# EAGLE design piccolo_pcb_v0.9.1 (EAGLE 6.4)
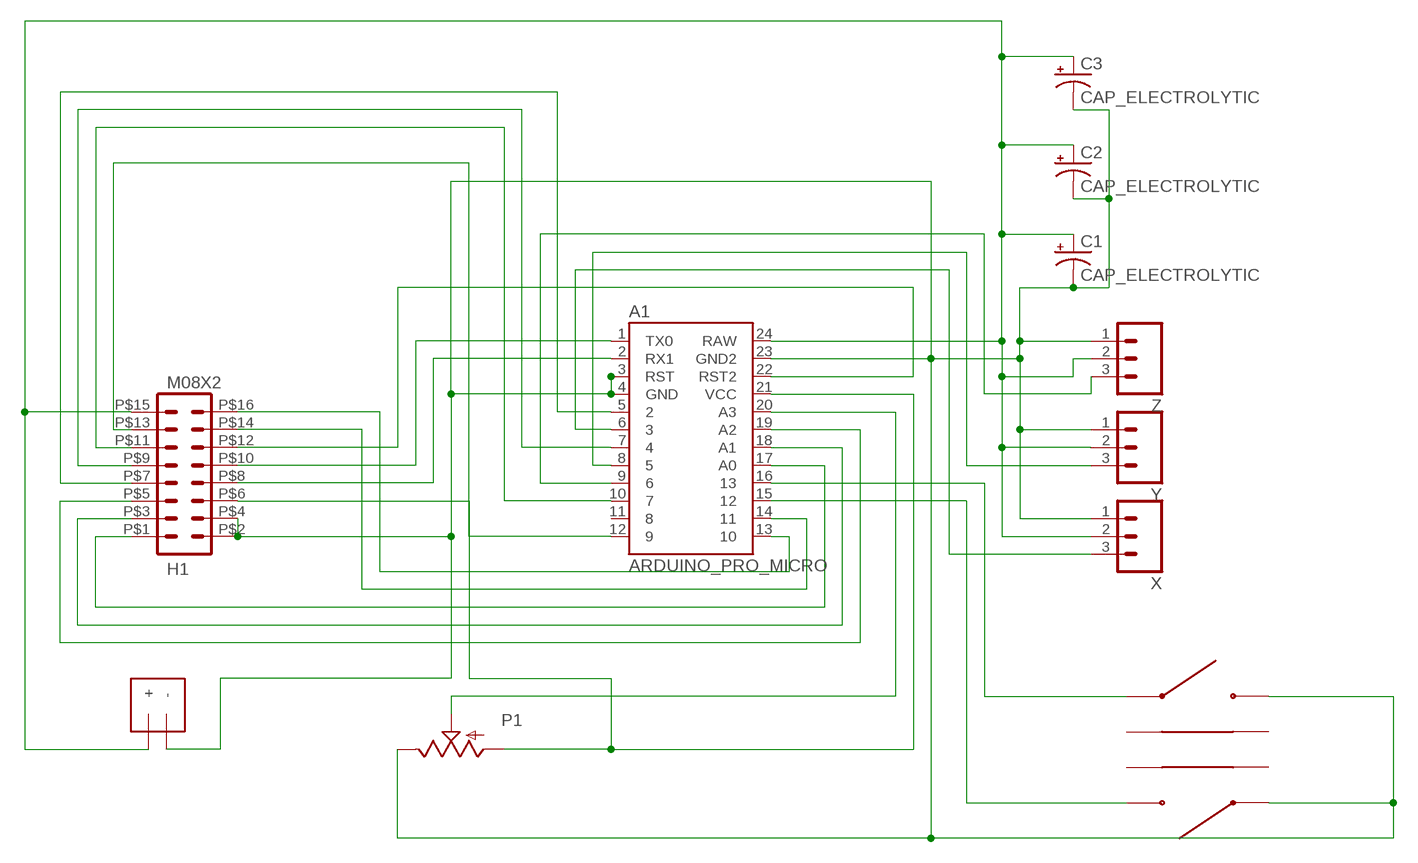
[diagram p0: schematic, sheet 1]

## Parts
A1  ARDUINO_PRO_MICRO  ARDUINO_MINI  [ARDUINO_MINI]
C1  CAP_ELECTROLYTIC  [RADIAL_330UF]
C2  CAP_ELECTROLYTIC  [RADIAL_330UF]
C3  CAP_ELECTROLYTIC  [RADIAL_330UF]
DC_IN  4.8v-6.0v  M02-POL  [JST-PH-2-PTH]
H1  M08X2  [PTH_2X8_90DEG_FEMALE]
P1  POTTHUMBWHEEL  [16MM_THUMBWHEEL]
S1  SWITCH_TACTILE  [RIGHT_ANGLE_TACTSWITCH]
S2  SWITCH_TACTILE  [RIGHT_ANGLE_TACTSWITCH]
X  M03PTH  [1X03]
Y  M03PTH  [1X03]
Z  M03PTH  [1X03]

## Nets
A3: A1.20(A3) P1.P$2(S)
GND: A1.3(RST) A1.4(GND) A1.23(GND2) C1.C(-) C2.C(-) C3.C(-) DC_IN.- H1.P$2 H1.P$4 P1.P$1(E) S1.1 S2.2 X.1 Y.1 Z.1
N$3: A1.15 S1.2
N$4: A1.16 S2.1
PIN2: A1.5 H1.P$7
PIN4: A1.7 H1.P$9
PIN7: A1.10 H1.P$11
PIN9: A1.12 H1.P$13
PIN10: A1.13 H1.P$16
PIN16: A1.14 H1.P$14
PIN_A0: A1.17(A0) H1.P$1
PIN_A1: A1.18(A1) H1.P$3
PIN_A2: A1.19(A2) H1.P$5
PWR_RAW: A1.24(RAW) C1.A(+) C2.A(+) C3.A(+) DC_IN.+ H1.P$15 X.2 Y.2 Z.2
RESET: A1.22(RST2) H1.P$12
RX: A1.2(RX1) H1.P$8
TX: A1.1(TX0) H1.P$10
VCC: A1.21(VCC) H1.P$6 P1.P$3(A)
X_PWM_PIN3: A1.6 X.3
Y_PWM_PIN5: A1.8 Y.3
Z_PWM_PIN6: A1.9 Z.3
Unconnected: A1.11 S1.PE1(GND1) S1.PE2(GND2) S2.PE1(GND1) S2.PE2(GND2)

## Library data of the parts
A1 = SparkFun-Boards:ARDUINO_MINI: Arduino Pro Mini footprint
C1-C3 = Piccolo:CAP_ELECTROLYTIC
DC_IN = Piccolo:M02-POL
H1 = Piccolo:M08X2
P1 = Piccolo:POT
S1 S2 = Piccolo:SWITCH_TACTILE
X Y Z = SparkFun-Connectors:M03: Header 3 Standard 3-pin 0.1" header. Use with straight break away headers (SKU : PRT-00116), right angle break away headers (PRT-00553), swiss pins (PRT-00743), machine pins (PRT-00117), and female headers (PRT-00115). Molex polarized connector foot print use with SKU : PRT-08232 with associated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

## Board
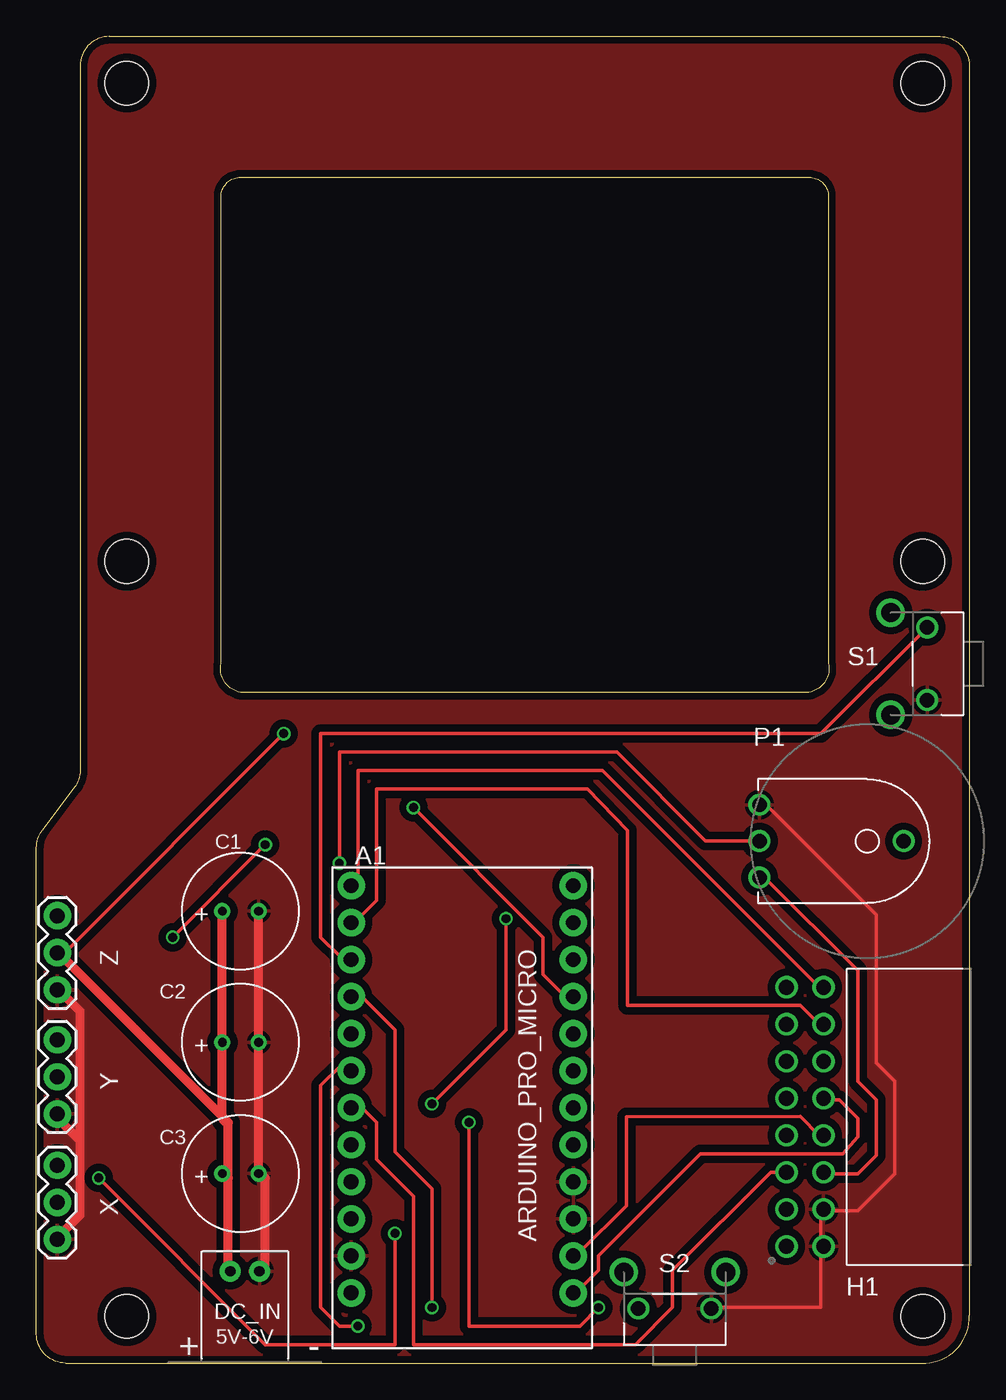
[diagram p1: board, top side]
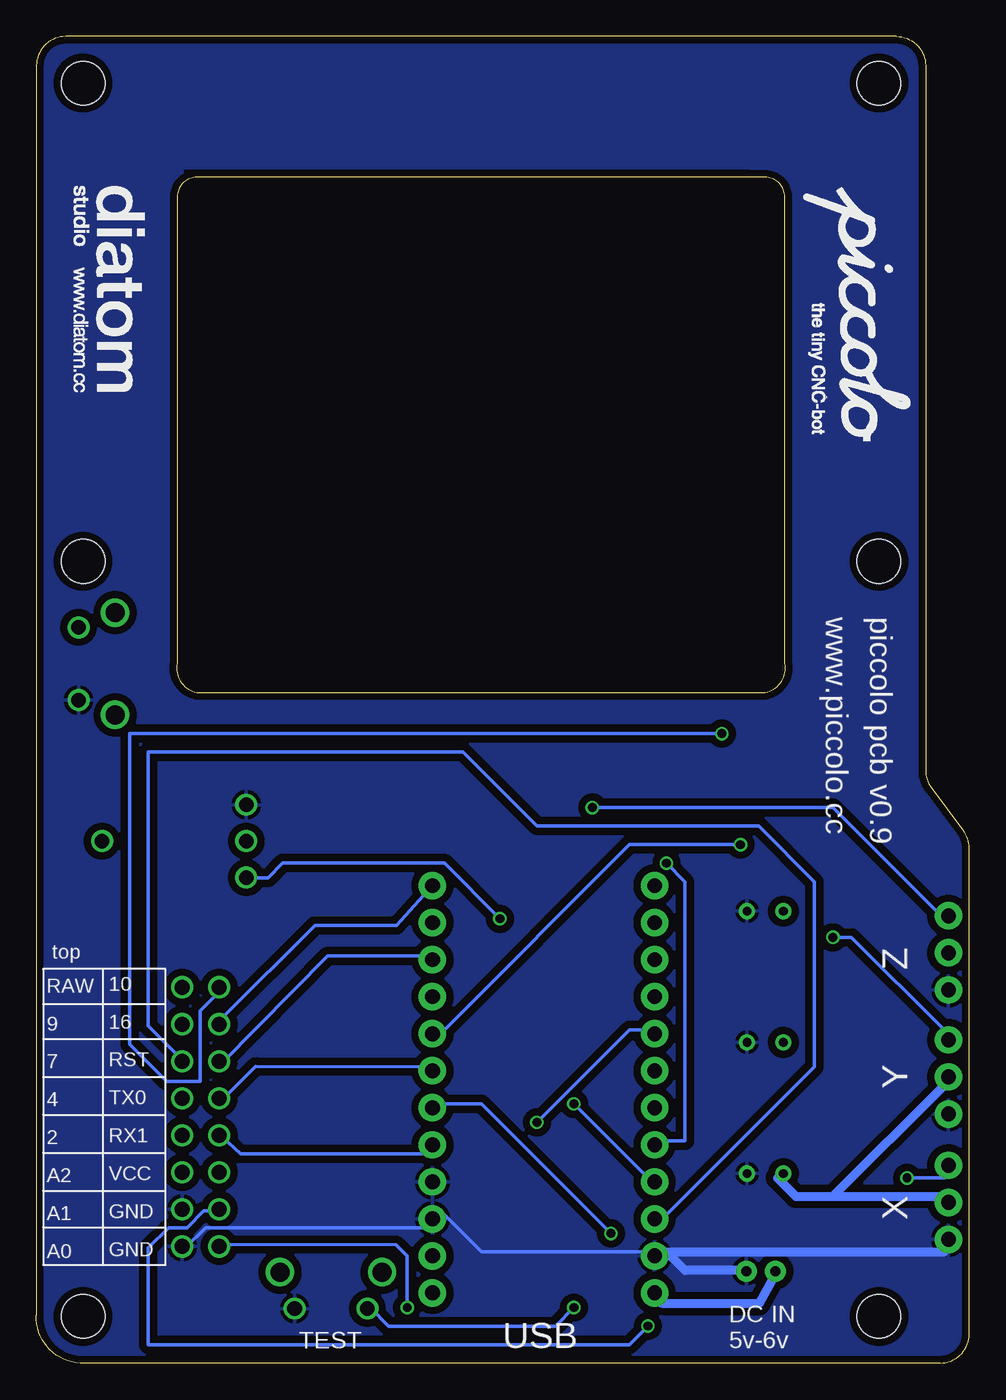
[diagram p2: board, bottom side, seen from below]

Size 64 x 91 mm. Coordinates in mm from the lower left corner, seen from the top.
Outline: 0,2 0,35.33 arc-37 0.4,36.53 2.6,39.47 arc37 3,40.67 3,89 arc-90 5,91 62,91 arc-90 64,89 64,3.27 arc-90 61,0 2,0 arc-90 0,2
Outline: 12.66,48 12.66,80 arc-90 14,81.34 53,81.34 arc-90 54.34,80 54.34,48 arc-90 53,46 14,46 arc-90 12.66,48
Copper layers (1*16): Top 0.035mm / dielectric 1.5mm / Bottom 0.035mm
Design rules "ITEADstudio_DRC": minimum track width 6mil, minimum drill 12mil, track to track 6mil, track to pad 6mil, pad to pad 6mil, via to via 6mil, smd to smd 0mil, copper to edge 10mil, drill to drill 10mil, minimum pad ring 10mil, minimum via ring 6mil, stop-mask expansion 2mil, vias tented up to drill 100mil, thermal gap 10mil
Holes 3 mm at 6.2,87.8 6.2,55 6.2,3.2 60.8,3.2 60.8,55 60.8,87.8

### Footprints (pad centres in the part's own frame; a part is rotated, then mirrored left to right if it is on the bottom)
ARDUINO_MINI = drill 1.016 pad 1.88: 1 -7.62,12.7; 2 -7.62,10.16; 3 -7.62,7.62; 4 -7.62,5.08; 5 -7.62,2.54; 6 -7.62,0; 7 -7.62,-2.54; 8 -7.62,-5.08; 9 -7.62,-7.62; 10 -7.62,-10.16; 11 -7.62,-12.7; 12 -7.62,-15.24; 13 7.62,-15.24; 14 7.62,-12.7; 15 7.62,-10.16; 16 7.62,-7.62; 17 7.62,-5.08; 18 7.62,-2.54; 19 7.62,0; 20 7.62,2.54; 21 7.62,5.08; 22 7.62,7.62; 23 7.62,10.16; 24 7.62,12.7
RADIAL_330UF = drill 0.6: A 0,1.25; C 0,-1.25
JST-PH-2-PTH = drill 0.7 pad 1.448: + -1,0; - 1,0
PTH_2X8_90DEG_FEMALE = drill 1.02: P$1 -2.54,0; P$2 0,0; P$3 -2.54,2.54; P$4 0,2.54; P$5 -2.54,5.08; P$6 0,5.08; P$7 -2.54,7.62; P$8 0,7.62; P$9 -2.54,10.16; P$10 0,10.16; P$11 -2.54,12.7; P$12 0,12.7; P$13 -2.54,15.24; P$14 0,15.24; P$15 -2.54,17.78; P$16 0,17.78
16MM_THUMBWHEEL = drill 1: P$1 -2.5,-7.4; P$2 0,-7.4; P$3 2.5,-7.4; P$4 0,2.5
RIGHT_ANGLE_TACTSWITCH = drill 1: 1 -2.5,0; 2 2.5,0 | drill 1.3: PE1 -3.5,2.5; PE2 3.5,2.5
1X03 = drill 1.016 pad 1.88: 1 0,0; 2 2.54,0; 3 5.08,0

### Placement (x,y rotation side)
A1  29.21,17.51 180 top
C1  14,31 90 top
C2  14,22 90 top
C3  14,13 90 top
DC_IN  14.3,6.3 0 top
H1  54,8 0 top
P1  57,35.8 270 top
S1  61.11,47.97 90 top
S2  43.79,3.74 0 top
X  1.43,8.48 90 top
Y  1.43,17.09 90 top
Z  1.43,25.6 90 top

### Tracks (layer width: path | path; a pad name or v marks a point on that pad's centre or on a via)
A3  (via drill 0.61)
  Top 0.254: v20.78,34.29 20.78,41.91 39.83,41.91 45.91,35.83 49.99,35.83 P1.P$2
  Bottom 0.254: v20.78,34.29 19.51,33.02 19.51,15.24 20.78,15.24 A1.20
GND
  Top 0.254: 53.8,7.89 53.8,3.81 46.18,3.81 S2.2 | 53.8,10.43 56.34,10.43 58.88,12.97 58.88,19.32 57.61,20.59 57.61,30.75 49.99,38.37 P1.P$1 | 53.8,10.43 53.8,7.89 | 53.8,7.89 H1.P$2 | 53.8,10.43 H1.P$4 | 1.73,8.89 X.1
  Top 0.61: DC_IN.- 15.7,6.35 15.7,12.7 C3.C C2.C C1.C | 3,15.24 1.73,16.51 Y.1 | 3,15.24 3,10.16 1.73,8.89 | 3,15.24 3,24.13 1.73,25.4 Z.1
  Bottom 0.254: A1.23 22.05,7.62 33.48,7.62 36.02,10.16 A1.3 37.42,9.27 52.4,9.29 53.8,7.89 H1.P$2
  Bottom 0.61: 20.78,7.62 19.51,6.35 15.7,6.35 DC_IN.- | 20.78,7.62 1.73,7.62 X.1 | 20.78,7.62 A1.23
  pour Bottom (isolate 0.5): 62,91 14,91 14,82 54,82 54,46 13,46 13,91 5,91 arc90 3,89 3,40 0,36 0,2 arc90 2,0 62,0 arc90 64,2 64,89 arc90
  pour Top (isolate 0.5): 62,91 54,91 54,46 13,46 13,91 5,91 arc90 3,89 3,40 0,36 0,2 arc90 2,0 62,0 arc90 64,3.27 64,90.27 arc90
  pour Bottom (isolate 0.5): 12,91 15,91 15,81 12,81
  pour Top (isolate 0.5): 13,91 54,91 54,81 13,81
N$3
  Top 0.254: A1.15 20.78,27.94 19.51,29.21 19.51,43.18 53.82,43.18 S1.2
N$4  (via drill 0.61)
  Top 0.254: v27.13,3.81 27.13,11.94 24.59,14.48 24.59,22.86 22.05,25.4 A1.16
  Bottom 0.254: v27.13,3.81 28.4,2.54 39.83,2.54 41.1,3.81 S2.1
PIN2
  Bottom 0.254: H1.P$7 51.26,15.51 49.99,14.37 37.54,14.35 A1.5
PIN4
  Bottom 0.254: H1.P$9 51.26,18.05 48.97,20.34 37.29,20.32 A1.7
PIN7
  Bottom 0.254: H1.P$11 51.26,20.59 44.02,27.94 37.29,27.94 A1.10
PIN9
  Bottom 0.254: 51.26,23.67 44.89,30.02 39.29,30.02 A1.12
  Bottom 0.61: H1.P$13 arc-90 51.26,23.44 51.26,23.67
PIN10
  Top 0.254: H1.P$16 53.8,25.67 38.83,40.64 22.05,40.64 22.05,33.02 A1.13
PIN16
  Top 0.254: H1.P$14 53.8,23.13 52.4,24.53 40.56,24.53 40.56,36.54 37.8,39.37 23.32,39.37 23.32,31.75 22.05,30.48 A1.14
PIN_A0  (via drill 0.61, 0.61 pad 0.66)
  Top 0.254: v38.56,3.81 37.29,2.54 29.67,2.54 v29.67,16.51
  Bottom 0.254: v38.56,3.81 38.56,7.37 39.32,8.13 51.01,8.14 51.26,7.89 H1.P$1 | v29.67,16.51 23.32,22.86 22.05,22.86 A1.17
PIN_A1  (via drill 0.61)
  Top 0.254: v22.05,2.54 20.78,2.54 19.51,3.81 19.51,19.05 20.78,20.32 A1.18
  Bottom 0.254: v22.05,2.54 23.32,1.27 56.34,1.27 56.34,7.89 54.94,9.29 53.67,9.29 52.53,10.43 51.26,10.43 H1.P$3
PIN_A2
  Top 0.254: H1.P$5 51.26,13.1 50.37,13.08 43.64,6.35 43.64,3.81 41.1,1.27 25.86,1.27 25.86,11.43 23.32,13.97 23.32,16.51 22.05,17.78 A1.19
PWR_RAW  (via drill 0.61)
  Top 0.254: 13.16,6.35 DC_IN.+ | Z.2 1.73,27.94 v16.97,43.18
  Top 0.61: 13.16,6.35 13.16,12.7 | 13.16,16.51 1.73,27.94 | 13.16,12.7 13.16,16.51 | 13.16,12.7 C3.A | 13.16,16.51 arc-90 12.75,16.92 C2.A C1.A
  Bottom 0.25: 52.78,24.15 51.26,25.67 H1.P$15
  Bottom 0.254: 13.16,12.7 C3.A | 13.16,6.35 DC_IN.+ | 1.73,19.05 Y.2 | 52.78,24.15 52.78,19.32 55.07,19.32 57.61,21.86 57.61,43.18 v16.97,43.18
  Bottom 0.61: 9.35,11.43 11.89,11.43 13.16,12.7 | 9.35,11.43 1.73,11.43 X.2 | 13.16,6.35 14.43,4.08 20.86,4.08 arc90 A1.24 | 9.35,11.43 1.73,19.05
RESET
  Bottom 0.254: H1.P$12 53.8,20.59 56.34,23.13 56.34,41.91 34.75,41.91 29.67,36.83 14.43,36.83 10.62,33.02 10.62,20.32 20.78,10.16 A1.22
RX
  Top 0.254: A1.2 37.29,7.62 40.47,10.79 40.47,16.89 52.4,16.91 53.69,15.62 H1.P$8
TX
  Top 0.254: A1.1 37.29,5.08 38.56,6.35 38.56,7.37 45.55,14.35 55.32,14.37 56.34,15.51 56.34,16.78 55.07,18.05 54.11,18.05 H1.P$10
VCC  (via drill 0.61)
  Top 0.254: P1.P$3 49.99,33.29 56.34,26.94 56.34,19.32 57.61,18.05 57.61,14.24 56.34,12.97 53.8,12.97 H1.P$6 | v27.13,17.78 32.21,22.86 v32.21,30.48
  Bottom 0.254: v27.13,17.78 22.05,12.7 A1.21 | v32.21,30.48 36.02,34.29 47.1,34.3 48.11,33.29 49.99,33.29 P1.P$3
X_PWM_PIN3  (via drill 0.61)
  Top 0.254: v4.27,12.7 15.7,1.27 24.59,1.27 v24.59,8.89
  Bottom 0.254: v4.27,12.7 1.73,12.7 X.3 | v24.59,8.89 33.48,17.78 36.02,17.78 A1.6
Y_PWM_PIN5  (via drill 0.61)
  Top 0.254: v15.7,35.56 v9.35,29.21
  Bottom 0.254: v9.35,29.21 8.08,29.21 1.73,22.86 Y.3 | v15.7,35.56 23.32,35.56 36.02,22.86 A1.8
Z_PWM_PIN6  (via drill 0.61)
  Top 0.254: v25.86,38.1 34.75,29.21 34.75,26.67 36.02,25.4 A1.9
  Bottom 0.254: v25.86,38.1 9.35,38.1 1.73,30.48 Z.3

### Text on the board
bPlace: C:/Users/BG/Downloads/diatom_logo_1bit.bmp | piccolo pcb v0.9 | www.piccolo.cc
bNames: Z | top | Y | X | 10 / 16 / RST / TX0 / RX1 / VCC / GND / GND | RAW / 9 / 7 / 4 / 2 / A2 / A1 / A0 | DC IN / 5v-6v | USB | TEST

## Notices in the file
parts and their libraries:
SparkFun-Boards: Licensing: CC v3.0 Share-Alike You are welcome to use this library for commercial purposes.
